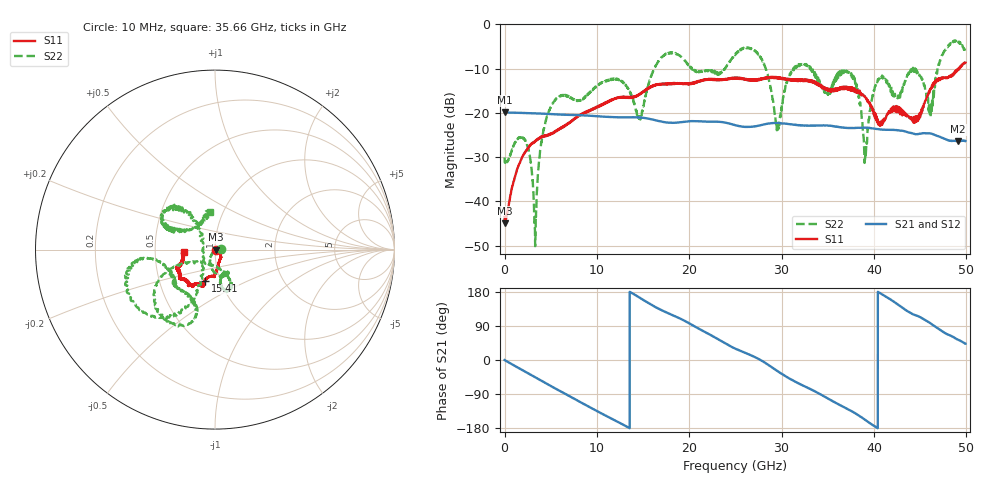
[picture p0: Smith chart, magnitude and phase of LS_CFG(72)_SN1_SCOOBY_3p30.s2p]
!Keysight Technologies,N5245B,MY58422026,A.13.80.08
!Date: Thursday, March 19, 2020 23:49:34
!Correction: S11(Full 2 Port(1,2))
!S21(Full 2 Port(1,2))
!S12(Full 2 Port(1,2))
!S22(Full 2 Port(1,2))
!S2P File: Measurements: S11, S21, S12, S22:
# Hz S DB R 50.0
!freq dBS11 angS11 dBS21 angS21 dBS12 angS12 dBS22 angS22
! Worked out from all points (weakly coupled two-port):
!   4991 points, 10 MHz to 49.91 GHz, reference 50 ohm
!   highest |S21| = -19.88 dB at 10 MHz (marker M1); lowest = -26.4 dB at 49.11 GHz (marker M2)
!   lowest |S11| = -45.0 dB at 40 MHz (marker M3), VSWR 1.01, Z = 50.6 + j0.00326 ohm
!   |S11| at or under -10 dB: start of sweep to 49.13 GHz; 49.16335 GHz to 49.2268 GHz (63.45 MHz wide, 0.129 % of centre)
!   |S22| runs from -50.1 to -3.6 dB; largest |S21 - S12| = 0.001
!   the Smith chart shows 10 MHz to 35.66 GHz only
!   S11 on the Smith chart (normalised r, x): 10 MHz: 1.01, -0.01; 15.41 GHz: 0.85, -0.31; 35.66 GHz: 0.70, -0.02
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1e7  -43.51 -24.9  -19.88 -0.2  -19.87 -0.3  -30.06 1.4
4e7  -44.99 0.3  -19.89 -0.6  -19.88 -0.7  -31.24 -3.9
2.18e9  -29.11 -39.0  -20.03 -30.1  -20.02 -30.0  -26.09 1.9
3.32e9  -26.31 -47.9  -20.11 -45.5  -20.10 -45.4  -50.11 -54.5
4.87e9  -24.80 -58.8  -20.25 -66.7  -20.24 -66.6  -19.35 -99.5
8.33e9  -20.43 -80.3  -20.54 -112.7  -20.53 -112.6  -17.03 -71.0
1.541e10  -14.71 -107.3  -21.23 152.9  -21.23 153.0  -15.10 -154.1
1.665e10  -13.61 -107.9  -21.81 135.8  -21.80 135.9  -8.37 -148.5
2.496e10  -12.21 -127.2  -22.73 30.3  -22.72 30.5  -6.90 -170.1
2.775e10  -12.26 -137.9  -22.79 -0.5  -22.78 -0.3  -7.36 -120.6
2.957e10  -11.92 -142.0  -22.29 -29.5  -22.28 -29.2  -23.07 -177.5
3.104e10  -12.52 -146.6  -22.60 -51.5  -22.60 -51.2  -10.74 130.2
3.328e10  -12.86 -156.4  -22.86 -78.9  -22.86 -78.5  -10.31 156.2
3.566e10  -15.11 -176.1  -22.99 -110.3  -22.93 -109.8  -13.11 98.1
3.781e10  -15.08 177.1  -23.42 -138.3  -23.37 -138.4  -11.94 135.3
3.905e10  -16.31 174.9  -23.34 -157.8  -23.33 -158.0  -30.34 -124.9
4.021e10  -21.34 163.9  -23.60 -176.8  -23.59 -177.0  -13.60 -5.1
4.16e10  -19.74 105.9  -23.82 162.9  -23.85 162.9  -13.78 25.2
4.445e10  -21.37 51.4  -24.80 118.6  -24.82 118.9  -10.15 -15.9
4.614e10  -14.56 5.8  -24.63 96.5  -24.64 96.6  -20.62 -46.9
4.911e10  -10.18 -14.4  -26.45 53.4  -26.47 53.6  -3.82 -44.6
4.991e10  -8.64 -14.5  -26.33 43.2  -26.35 43.3  -6.18 -29.4
